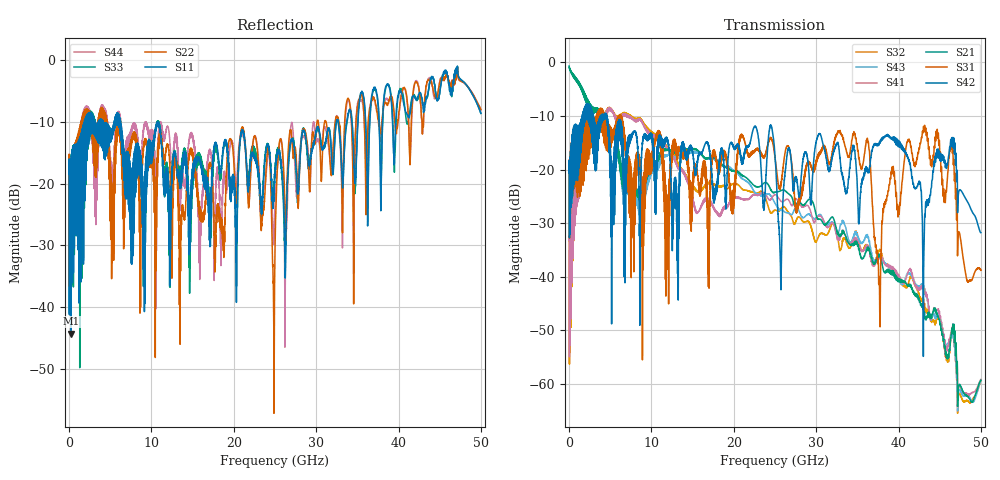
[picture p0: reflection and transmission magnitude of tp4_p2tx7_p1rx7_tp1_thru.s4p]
! 100G CR Analysis
! File: tp4_p2tx7_p1rx7_tp1_thru
! Description: 2m Cu Cable, OSFP, TP1-TP4
! Port Mapping
! Port1 -- P1RX7N
! Port2 -- P2TX7N
! Port3 -- P1RX7P
! Port4 -- P2TX7P
# GHz S MA R 50.00
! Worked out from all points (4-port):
!   5000 points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, 10 MHz to 50 GHz, reference 50 ohm
!   strongest paths, dB at 10 MHz, 12.51 GHz, 25.01 GHz, 37.51 GHz, 50 GHz:
!     S42: -20.5, -27.3, -17.5, -15.5, -31.8
!     S31: -20.5, -15.9, -17.8, -36.7, -38.8
!     S21: -0.7, -16.8, -24.2, -36.3, -59.3
!     S41: -33.2, -17.3, -24.7, -36.8, -59.2
!     S43: -0.7, -17.8, -26.3, -36.9, -59.2
!     S32: -33.3, -16.7, -27.6, -35.7, -59.4
!   lowest |S11| = -44.2 dB at 260 MHz (marker M1), VSWR 1.01, Z = 50.4 + j0.49 ohm
!   |S11| at or under -10 dB: start of sweep to 1.887 GHz; 4.132 GHz to 5.497 GHz (1.365 GHz wide, 28.4 % of centre); 6.252 GHz to 32.45 GHz (26.2 GHz wide, 135 % of centre)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
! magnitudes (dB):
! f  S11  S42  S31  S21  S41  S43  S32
! 10 MHz  -18.4  -20.5  -20.5  -0.7  -33.2  -0.7  -33.3
! 260 MHz  -44.2  -27.1  -26.2  -1.7  -47.8  -1.7  -49.4
! 6.86 GHz  -22.4  -30.4  -16.8  -23.1  -9.6  -23.8  -9.4
! 34.62 GHz  -17.2  -16.4  -13.4  -34.0  -33.1  -32.3  -32.2
! 37.65 GHz  -10.4  -15.3  -41.5  -36.1  -36.6  -36.7  -35.3
! 43.21 GHz  -6.9  -28.9  -12.9  -47.9  -43.1  -43.2  -46.2
! 50 GHz  -8.7  -31.8  -38.8  -59.3  -59.2  -59.2  -59.4
